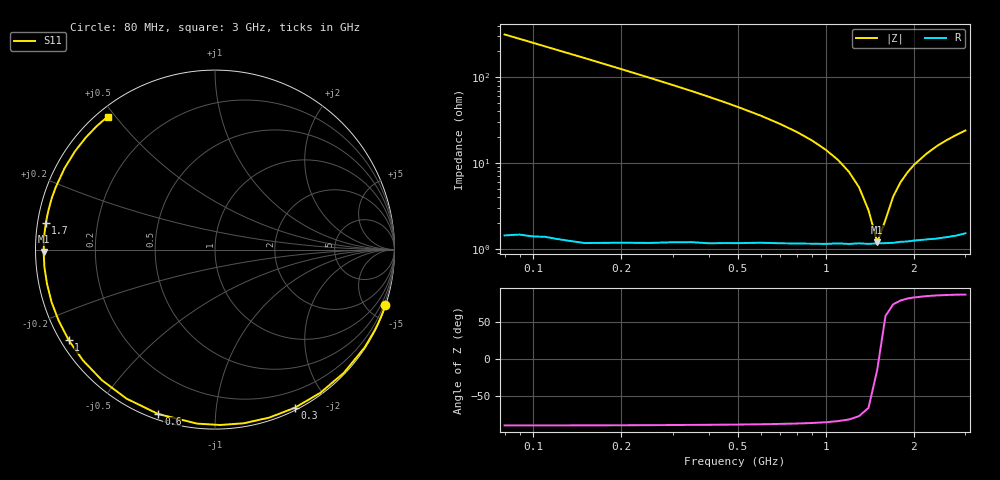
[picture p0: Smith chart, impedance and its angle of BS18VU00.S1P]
! SIEMENS Small Signal Semiconductors
! BB640
! Si Tuning Diode in SOD323
! VR = 18 V
! S-Parameters:  July  1993
# GHz  S  MA  R  50
!  f  S11
! GHz  MAG  ANG
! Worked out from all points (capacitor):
!   33 points, 80 MHz to 3 GHz, reference 50 ohm
!   read as one part to ground: C = 6.28 pF near 80 MHz
!   lowest |Z| = 1.2 ohm at 1.5 GHz (marker M1)
!   series resonance near 1.514 GHz, so ESL is about 1.8 nH
!   S11 on the Smith chart (normalised r, x): 80 MHz: 0.03, -6.31; 300 MHz: 0.02, -1.63; 600 MHz: 0.02, -0.71; 1 GHz: 0.02, -0.28; 1.7 GHz: 0.02, +0.08; 3 GHz: 0.03, +0.48
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0.08  0.9986 -18.0
0.11  0.9975 -24.6
0.15  0.9962 -33.2
0.2  0.9935 -43.7
0.25  0.9905 -53.7
0.3  0.987 -63.2
0.35  0.9836 -72.1
0.4  0.9808 -80.6
0.45  0.9776 -88.4
0.5  0.9747 -95.8
0.6  0.9693 -109.0
0.7  0.9656 -120.7
0.8  0.9626 -130.9
0.9  0.9603 -140.0
1  0.9587 -148.2
1.1  0.9568 -155.5
1.2  0.9565 -162.2
1.4  0.9555 -174.1
1.5  0.9548 -179.3
1.6  0.9546 175.8
1.7  0.9544 171.1
1.8  0.9535 166.7
2  0.953 158.7
2.2  0.9529 151.6
2.4  0.9532 145.0
2.6  0.953 139.2
2.8  0.9528 133.8
3  0.9519 128.9
